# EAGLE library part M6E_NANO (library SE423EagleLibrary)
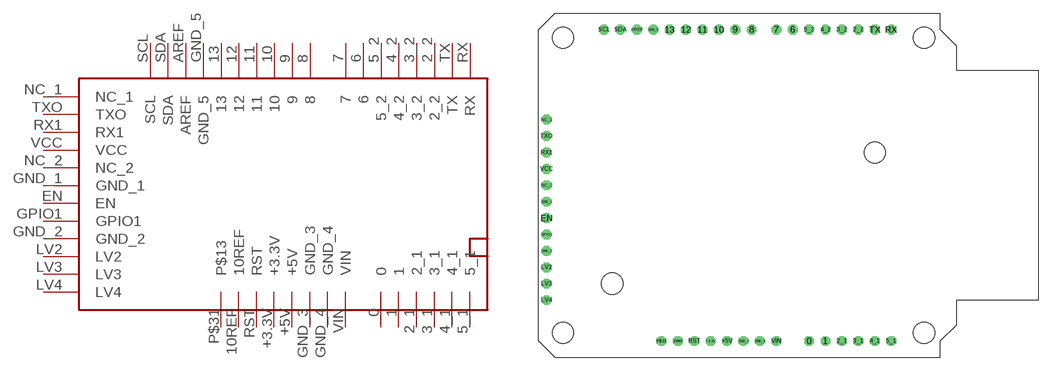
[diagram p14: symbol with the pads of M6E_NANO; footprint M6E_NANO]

Designator prefix -

## M6E_NANO  [M6E_NANO]
0  0
1  1
2_1  2_1
2_2  2_2
3_1  3_1
3_2  3_2
4_1  4_1
4_2  4_2
5_1  5_1
5_2  5_2
6  6
7  7
8  8
9  9
10  10
10REF  10REF
11  11
12  12
13  13
+3.3V  +3.3V
+5V  +5V
AREF  AREF
EN  EN
GND_1  GND_1
GND_2  GND_2
GND_3  GND_3
GND_4  GND_4
GND_5  GND_5
GPIO1  GPIO1
LV2  LV2
LV3  LV3
LV4  LV4
NC_1  NC_1
NC_2  NC_2
P$31  P$13
RST  RST
RX  RX
RX1  RX1
SCL  SCL
SDA  SDA
TX  TX
TXO  TXO
VCC  VCC
VIN  VIN

## Footprint M6E_NANO (pad centres in mm)
drill 1.016 octagon: 0 41.91,2.54; 1 44.45,2.54; 2_1 46.99,2.54; 2_2 49.53,50.8; 3_1 49.53,2.54; 3_2 46.99,50.8; 4_1 52.07,2.54; 4_2 44.45,50.8; 5_1 54.61,2.54; 5_2 41.91,50.8; 6 39.37,50.8; 7 36.83,50.8; 8 33.02,50.8; 9 30.48,50.8; 10 27.94,50.8; 10REF 21.59,2.54; 11 25.4,50.8; 12 22.86,50.8; 13 20.32,50.8; +3.3V 26.67,2.54; +5V 29.21,2.54; AREF 15.24,50.8; EN 1.27,21.59; GND_1 1.27,24.13; GND_2 1.27,16.51; GND_3 31.75,2.54; GND_4 34.29,2.54; GND_5 17.78,50.8; GPIO1 1.27,19.05; LV2 1.27,13.97; LV3 1.27,11.43; LV4 1.27,8.89; NC_1 1.27,36.83; NC_2 1.27,26.67; P$31 19.05,2.54; RST 24.13,2.54; RX 54.61,50.8; RX1 1.27,31.75; SCL 10.16,50.8; SDA 12.7,50.8; TX 52.07,50.8; TXO 1.27,34.29; VCC 1.27,29.21; VIN 36.83,2.54
hole 3.302 at 3.81,3.81
hole 3.302 at 11.43,11.43
hole 3.302 at 3.81,49.53
hole 3.302 at 59.69,49.53
hole 3.302 at 59.69,3.81
hole 3.302 at 52.07,31.75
